(* 	This implementation of user defined system clock is only for demonstration purposes. 
	Real application use some high resolution time source (e.g. GPS clock). *)
FUNCTION_BLOCK FB_MyClock IMPLEMENTS I_ScsmSystemClockEventSink
VAR
	_tT : T_UtcTime:=(secondSinceEpoch:=DT#2021-04-01-00:00:00, quality:=(ClockNotSynchronized:=TRUE, ClockFailure:=FALSE, LeapSecondsKnown:=FALSE), fractionOfSecond:=[0,0,0]);(* Actual UTC time. *)
	_tB : T_BinaryTime;(* Actual binary-time (EntryTime) *)
	clock : RTC_EX:=(EN:=TRUE, PDT:=DT#2021-04-01-00:00:00, PMSEK:=0);
	refreshTimer : TON:=(IN:=TRUE, PT:=T#1S);
END_VAR

METHOD FINAL Execute : BOOL
refreshTimer();
IF Execute:=refreshTimer.Q THEN
	refreshTimer(IN:=FALSE); refreshTimer(IN:=TRUE);
	Update();
END_IF
END_METHOD

(* This method is called every time the ied needs actual time. Return value: TRUE => success, returned time is valid, FALSE => failure. *)
METHOD FINAL OnGetSystemTime : BOOL
VAR_INPUT
	ipAA: I_ScsmAssociationClass;(* Application association. If = 0 => optional or unknown. *)
END_VAR
VAR_OUTPUT
	tT: T_UtcTime;(* UTC-time. *)
	tB: T_BinaryTime;(* Binary-time *)
END_VAR
tT:=_tT;
tB:=_tB;
OnGetSystemTime:=TRUE;
END_METHOD

(* This method sets clock time. *)
METHOD FINAL SetClock
VAR_INPUT
	tSet : DT;(* New time to set *)
END_VAR
clock(EN:=FALSE);
clock(EN:=TRUE, PDT:=tSet);
_tT.quality.ClockNotSynchronized:=FALSE;
Update();
END_METHOD

METHOD FINAL Update
clock();(* update clock time *)

(* convert to utc-time format *)
_tT.secondSinceEpoch:=clock.CDT;
_tT.fractionOfSecond:=LTIME_TO_UtcTimeFractionofSecond(in:=TIME_TO_LTIME(DWORD_TO_TIME(clock.CMSEK)));
Accuracy_To_UtcTimeQualityAccuracy(in:=E_UtcTimeAccuracy._03, bAccuracy0=>_tT.quality.Accuracy0, bAccuracy1=>_tT.quality.Accuracy1, bAccuracy2=>_tT.quality.Accuracy2, bAccuracy3=>_tT.quality.Accuracy3, bAccuracy4=>_tT.quality.Accuracy4);

(* convert to binary-time format *)
_tB.day:=Date_To_BinaryTime6Day(in:=DT_TO_DATE(clock.CDT));
_tB.timeOfDay:=DT_TO_TOD(clock.CDT) + DWORD_TO_TIME(clock.CMSEK);
END_METHOD

END_FUNCTION_BLOCK
